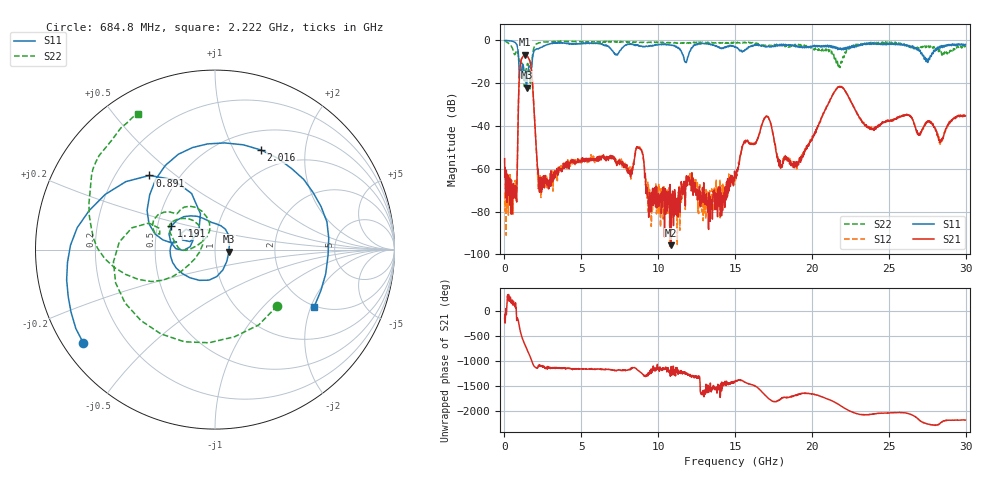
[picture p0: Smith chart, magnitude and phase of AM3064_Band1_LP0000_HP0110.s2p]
# Hz S DB R 50.0
!freq dBS11 angS11 dBS21 angS21 dBS12 angS12 dBS22 angS22
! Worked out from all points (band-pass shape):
!   1600 points, 10 MHz to 29.98 GHz, reference 50 ohm
!   highest |S21| = -6.74 dB at 1.341 GHz (marker M1); lowest = -95.8 dB at 10.84 GHz (marker M2)
!   |S21| within 3 dB of the highest: 1.071 GHz to 1.656 GHz (585 MHz wide, 42.9 % of centre)
!   lowest |S11| = -22.1 dB at 1.435 GHz (marker M3), VSWR 1.17, Z = 58.4 - j1.27 ohm
!   |S11| at or under -10 dB: 931.3 MHz to 1.799 GHz (867.4 MHz wide, 63.5 % of centre); 11.74 GHz to 11.84 GHz (102 MHz wide, 0.865 % of centre); 27.52159 GHz to 27.55064 GHz (29.05 MHz wide, 0.105 % of centre)
!   |S22| runs from -22.6 to -0.2 dB; largest |S21 - S12| = 0.0053
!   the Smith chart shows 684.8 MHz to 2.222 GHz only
!   S11 on the Smith chart (normalised r, x): 684.8 MHz: 0.06, -0.32; 891 MHz: 0.34, +0.41; 1.191 GHz: 0.59, +0.17; 2.016 GHz: 0.73, +1.29; 2.222 GHz: 1.94, -2.11
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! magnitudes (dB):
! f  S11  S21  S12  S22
! 10 MHz  0.0  -55.3  -71.4  -0.2
! 684.8 MHz  -0.9  -67.6  -67.4  -6.6
! 891 MHz  -5.2  -35.9  -35.9  -6.4
! 1.191 GHz  -11.2  -7.6  -7.6  -11.7
! 1.341 GHz  -16.9  -6.7  -6.7  -17.4
! 1.435 GHz  -22.1  -7.0  -7.0  -12.6
! 1.734 GHz  -13.2  -12.5  -12.4  -15.5
! 2.016 GHz  -4.3  -43.5  -43.8  -2.1
! 2.222 GHz  -3.9  -68.9  -64.9  -1.2
! 5.015 GHz  -1.4  -56.6  -55.5  -0.8
! 8.763 GHz  -2.6  -50.2  -50.2  -1.0
! 9.401 GHz  -2.5  -75.7  -82.8  -0.8
! 10 GHz  -2.0  -76.7  -69.5  -0.9
! 10.84 GHz  -2.2  -95.8  -80.0  -1.0
! 15 GHz  -3.1  -61.7  -62.1  -1.3
! 17.01 GHz  -3.1  -35.5  -35.5  -2.5
! 17.93 GHz  -2.1  -59.2  -57.1  -1.9
! 19.99 GHz  -3.1  -46.3  -46.2  -3.4
! 21.79 GHz  -4.1  -21.5  -21.6  -11.9
! 25 GHz  -1.3  -37.6  -37.6  -1.0
! 28.39 GHz  -2.7  -47.3  -46.6  -5.2
! 29.98 GHz  -1.9  -35.3  -34.9  -3.2
